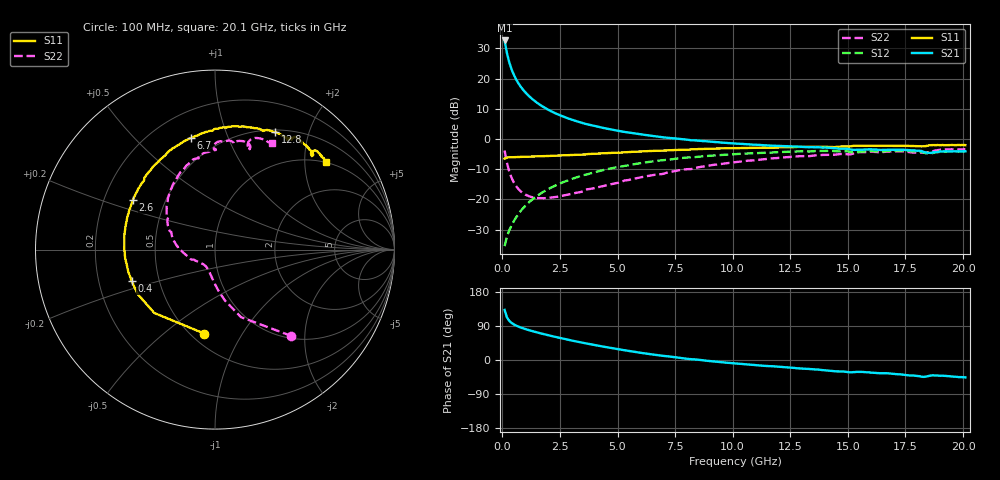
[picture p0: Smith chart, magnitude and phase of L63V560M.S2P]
!  Infineon Technologies AG
! BFR380L3 , PF131585-7, No.6, Th 09.10.01, soldered on pcb-board, measured with PP GSG850
!  Vce=3.5 V,  Ic=60.0 mA
! Common Emitter S-Parameters:  15. November 2001
#  GHz  S  MA  R  50
! f  S11  S21  S12  S22
! GHz  Mag  Ang  Mag  Ang  Mag  Ang  Mag  Ang
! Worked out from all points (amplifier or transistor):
!   201 points, 100 MHz to 20.1 GHz, reference 50 ohm
!   highest |S21| = 32.6 dB at 100 MHz (marker M1)
!   |S21| within 3 dB of that: start of sweep to 172.2 MHz
!   unconditionally stable (mu >= 1): 835.3 MHz to 4.216 GHz; 18.37595 GHz to 18.44419 GHz
!   at 3.4 GHz: K = 1.02, MAG = 8.0 dB, |S12| = -12.3 dB
!   at 10.1 GHz: K = 0.95, MSG = 1.8 dB, |S12| = -5.0 dB
!   at 20.1 GHz: K = 0.99, MSG = 0.0 dB, |S12| = -4.1 dB
!   S11 on the Smith chart (normalised r, x): 100 MHz: 0.58, -0.70; 400 MHz: 0.35, -0.16; 2.6 GHz: 0.32, +0.25; 6.7 GHz: 0.36, +0.75; 12.8 GHz: 0.52, +1.51; 20.1 GHz: 0.99, +2.56
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0.1  0.4717 -97.2  42.65 132.2  0.01676 60.2  0.6412 -48.5
0.2  0.489 -133.8  26.44 112.6  0.02418 58.4  0.4035 -68.9
0.3  0.4966 -149.9  18.62 103.5  0.03065 61.1  0.2897 -78.9
0.4  0.4964 -159.5  14.28 97.9  0.03687 63.3  0.2279 -85.5
0.5  0.4984 -165.9  11.54 93.9  0.0435 65.7  0.1899 -90.5
0.6  0.499 -170.6  9.68 90.8  0.05033 67.1  0.1653 -94.6
0.7  0.503 -174.5  8.345 88.1  0.05706 68.3  0.1478 -98.4
0.8  0.5033 -177.7  7.325 85.7  0.06428 69.1  0.1354 -101.8
1  0.5055 176.8  5.901 81.6  0.07803 69.7  0.1196 -107.8
1.3  0.5117 170.5  4.571 76.2  0.09904 69.6  0.1083 -115.9
1.6  0.5157 164.7  3.744 71.3  0.1203 68.7  0.1047 -122.9
2  0.522 158.0  3.032 65.3  0.1481 66.9  0.1056 -131.3
2.6  0.5343 148.9  2.378 56.9  0.1893 63.6  0.1147 -142.6
3.5  0.5507 136.5  1.824 45.2  0.2497 57.6  0.1351 -155.8
5.1  0.5927 118.1  1.345 27.5  0.3485 46.2  0.1906 -178.9
6.7  0.6369 102.0  1.099 13.1  0.432 35.1  0.2576 160.2
6.8  0.6395 101.0  1.086 12.3  0.4375 34.3  0.2605 159.0
10.1  0.7041 76.8  0.8383 -8.9  0.5596 12.2  0.4117 127.2
12.8  0.7375 62.8  0.7456 -21.9  0.6198 -4.7  0.5155 104.1
13.5  0.7385 59.3  0.7277 -24.5  0.6252 -8.8  0.5287 99.4
16.8  0.7694 47.2  0.6616 -35.5  0.631 -24.9  0.6183 78.1
20.1  0.789 38.1  0.6245 -45.9  0.624 -38.6  0.6742 61.7
